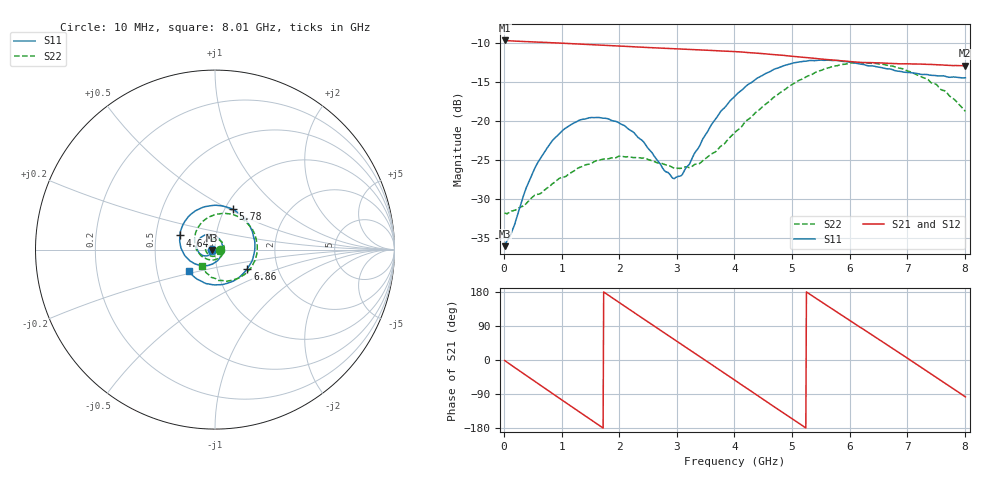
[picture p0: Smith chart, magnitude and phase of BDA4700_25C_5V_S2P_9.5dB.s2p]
!Agilent Technologies,E5071B,MY42404982,A.09.10
!Date: Mon Oct 20 13:30:48 2025
!Data & Calibration Information:
!Freq	S11:SOLT2(ON)	S21:SOLT2(ON)	S12:SOLT2(ON)	S22:SOLT2(ON)
# Hz S RI R 50
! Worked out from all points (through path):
!   801 points, 10 MHz to 8.01 GHz, reference 50 ohm
!   highest |S21| = -9.62 dB at 10 MHz (marker M1); lowest = -12.9 dB at 8 GHz (marker M2)
!   group delay of S21, straight-line fit = 283 ps
!   lowest |S11| = -36.0 dB at 10 MHz (marker M3), VSWR 1.03, Z = 48.5 - j0.133 ohm
!   |S11| at or under -10 dB: start of sweep to end of sweep
!   |S22| runs from -31.9 to -12.5 dB; largest |S21 - S12| = 0.0025
!   S11 on the Smith chart (normalised r, x): 10 MHz: 0.97, -0.00; 4.64 GHz: 0.67, +0.11; 5.78 GHz: 1.09, +0.52; 6.86 GHz: 1.40, -0.31; 8.01 GHz: 0.72, -0.18
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1e7  -0.0157 -0.00138  0.3301 -0.00711  0.3302 -0.00766  0.0258 -0.0014
3.3e8  -0.0237 -0.0223  0.2662 -0.1869  0.2661 -0.1873  0.0217 -0.0184
7.2e8  -0.0545 -0.0352  0.0781 -0.311  0.0784 -0.3111  -0.00105 -0.0365
1.02e9  -0.0846 -0.022  -0.0931 -0.303  -0.0932 -0.3032  -0.0281 -0.0334
1.35e9  -0.1018 0.014  -0.2441 -0.1956  -0.2442 -0.1957  -0.0507 -0.0062
1.93e9  -0.0611 0.0792  -0.2845 0.1101  -0.2846 0.1102  -0.0252 0.0525
2.32e9  -0.00493 0.079  -0.1448 0.2625  -0.1448 0.2626  0.021 0.0545
2.68e9  0.0355 0.0422  0.0403 0.2928  0.0402 0.2928  0.0497 0.0209
2.93e9  0.043 0.00202  0.1607 0.2445  0.1608 0.2441  0.0495 -0.00929
3.07e9  0.0389 -0.0219  0.2152 0.1959  0.2143 0.1968  0.0423 -0.0264
3.53e9  -0.0208 -0.0827  0.2848 -0.0224  0.285 -0.0228  -0.00933 -0.058
4.01e9  -0.1261 -0.0713  0.166 -0.2254  0.1662 -0.2252  -0.0777 -0.0339
4.64e9  -0.1952 0.079  -0.1273 -0.2365  -0.127 -0.2369  -0.1101 0.0828
5e9  -0.1499 0.1813  -0.2366 -0.1107  -0.2373 -0.111  -0.0657 0.159
5.35e9  -0.0501 0.2402  -0.2501 0.0462  -0.2504 0.0456  0.0225 0.1987
5.78e9  0.0996 0.2248  -0.1459 0.1981  -0.1455 0.1981  0.1483 0.172
6.21e9  0.2028 0.1132  0.0254 0.2372  0.0277 0.2373  0.2288 0.0627
6.68e9  0.2107 -0.051  0.188 0.1415  0.1886 0.1415  0.213 -0.0792
6.86e9  0.1803 -0.1067  0.2211 0.0766  0.2215 0.0754  0.181 -0.1238
7.35e9  0.0423 -0.1949  0.2003 -0.1167  0.2003 -0.1172  0.0595 -0.1763
8e9  -0.1448 -0.1228  -0.0252 -0.2256  -0.0252 -0.2261  -0.0726 -0.0916
8.01e9  -0.1471 -0.1205  -0.0294 -0.2251  -0.029 -0.2255  -0.0737 -0.0892
